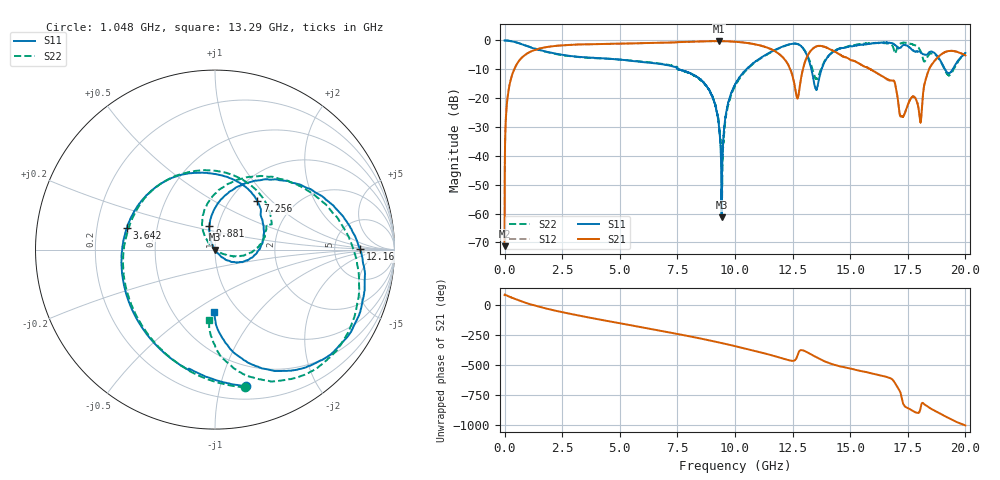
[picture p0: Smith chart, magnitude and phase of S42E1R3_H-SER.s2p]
!{S42E1R3}
!Johanson Technology Inc.
!www.johansontechnology.com
!Test Board Conditions:
!Substrate Type  RO4350B
!Substrate Thickness  50 mil
!Substrate Dk  3.66
!TL Type: GCPW
!TL Trace Width  60 mil
!TL Gap  10 mil
!Electrode orientation  Horizontal
!DUT TOPOLOGY	SERIES
!Mounting Pad LxW  14x55 mil
! Created Wed Nov 25 21:33:28 2020
# khz S ma R 50
! 2 Port Network Data from SP1.SP block
! freq  magS11  angS11  magS21  angS21  magS12  angS12  magS22  angS22
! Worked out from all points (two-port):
!   20001 points, 300 kHz to 20 GHz, reference 50 ohm
!   highest |S21| = -0.22 dB at 9.299 GHz (marker M1); lowest = -71.3 dB at 300 kHz (marker M2)
!   |S21| within 3 dB of the highest: 1.337 GHz to 11.62 GHz (10.28 GHz wide, 159 % of centre); 13.33 GHz to 14.16 GHz (832.5 MHz wide, 6.06 % of centre)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
!   lowest |S11| = -61.3 dB at 9.42 GHz (marker M3), VSWR 1.00, Z = 50.1 + j0.0219 ohm
!   |S11| at or under -10 dB: 7.537 GHz to 10.49 GHz (2.956 GHz wide, 32.8 % of centre); 13.31 GHz to 13.76 GHz (442.4 MHz wide, 3.27 % of centre); 19.11 GHz to 19.44 GHz (331.4 MHz wide, 1.72 % of centre)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
!   |S22| runs from -56.6 to 0.0 dB; largest |S21 - S12| = 0.012
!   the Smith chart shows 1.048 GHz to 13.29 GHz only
!   S11 on the Smith chart (normalised r, x): 1.048 GHz: 0.31, -1.20; 3.642 GHz: 0.33, +0.11; 7.256 GHz: 1.32, +0.83; 9.881 GHz: 0.91, +0.24; 12.16 GHz: 9.39, +0.20; 13.29 GHz: 0.78, -0.61
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300  0.9995 -0.2  0.0002726 84.9  0.0002778 106.0  1 -0.3
104300  0.9949 -8.8  0.08416 80.9  0.08459 80.9  0.9963 -8.8
207300  0.9841 -17.3  0.1649 72.1  0.1656 72.0  0.9844 -17.4
1048300  0.7787 -77.4  0.6179 12.6  0.6169 12.6  0.7853 -77.8
3334300  0.5162 178.1  0.8541 -89.6  0.8535 -89.6  0.5114 -177.6
3642300  0.5065 166.3  0.8582 -101.1  0.8595 -101.1  0.4984 171.3
6667300  0.3952 69.0  0.9117 151.0  0.9101 150.9  0.4018 54.4
7256300  0.3596 49.1  0.9224 129.7  0.9216 129.7  0.3668 32.9
8719300  0.1709 -23.6  0.9667 74.4  0.9661 74.4  0.1695 -10.3
9299300  0.0346 -50.1  0.9753 50.3  0.9746 50.2  0.03894 -29.4
9420300  0.0008564 14.8  0.9719 45.1  0.9736 45.0  0.005978 -21.3
9881300  0.1352 103.3  0.957 24.9  0.9559 24.9  0.1277 122.5
1.00003e7  0.1721 98.4  0.9491 19.6  0.9488 19.6  0.1622 116.5
1.21563e7  0.8076 0.3  0.4665 -88.3  0.4737 -87.8  0.8033 -7.5
1.27113e7  0.8697 -42.0  0.09814 -58.5  0.1008 -58.6  0.866 -51.1
1.32923e7  0.3442 -91.3  0.6663 -48.2  0.6659 -48.1  0.391 -94.4
1.33343e7  0.2936 -92.1  0.6936 -52.7  0.6948 -52.7  0.3442 -94.3
1.43773e7  0.677 -48.4  0.6252 -139.7  0.6294 -139.8  0.6824 -58.4
1.66673e7  0.911 -144.7  0.2089 117.8  0.2046 119.2  0.891 -160.2
1.80283e7  0.6384 165.6  0.04283 -159.5  0.04505 -159.5  0.685 135.7
1.90593e7  0.35 130.5  0.6117 161.0  0.6119 161.0  0.3386 118.4
2e7  0.6049 162.2  0.5504 77.9  0.5506 78.8  0.5982 142.9
